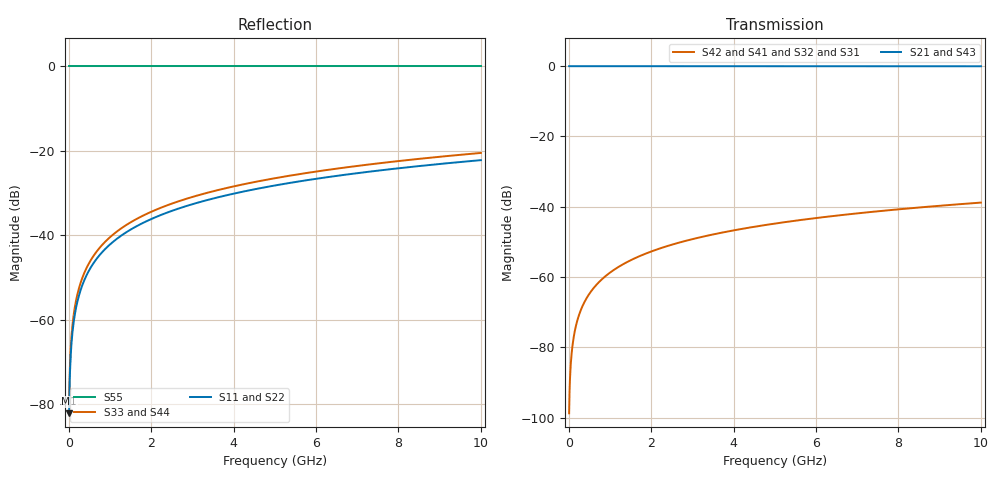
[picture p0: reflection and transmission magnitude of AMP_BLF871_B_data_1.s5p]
! Created Mon Feb  8 16:41:15 2010
# ghz S ma R 50
! 5 Port Network Data from SP1.SP block
! freq  magS11  angS11  magS12  angS12  magS13  angS13  magS14  angS14
!  magS15  angS15
!  magS21  angS21  magS22  angS22  magS23  angS23
!  magS24  angS24  magS25  angS25
!  magS31  angS31  magS32  angS32
!  magS33  angS33  magS34  angS34  magS35  angS35
!  magS41  angS41
!  magS42  angS42  magS43  angS43  magS44  angS44  magS45  angS45
!  magS51  angS51  magS52  angS52  magS53  angS53  magS54  angS54
!  magS55  angS55
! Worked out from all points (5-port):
!   1000 points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, 10 MHz to 10 GHz, reference 50 ohm
!   strongest paths, dB at 10 MHz, 2.51 GHz, 5.01 GHz, 7.51 GHz, 10 GHz:
!     S21: 0.0, 0.0, 0.0, 0.0, 0.0
!     S43: 0.0, 0.0, 0.0, 0.0, 0.0
!     S42: -98.7, -50.7, -44.8, -41.3, -38.8
!     S41: -98.7, -50.7, -44.8, -41.3, -38.8
!     S32: -98.7, -50.7, -44.8, -41.3, -38.8
!     S31: -98.7, -50.7, -44.8, -41.3, -38.8
!   lowest |S11| = -82.2 dB at 10 MHz (marker M1), VSWR 1.00, Z = 50 + j0.00776 ohm
!   |S11| at or under -10 dB: start of sweep to end of sweep
